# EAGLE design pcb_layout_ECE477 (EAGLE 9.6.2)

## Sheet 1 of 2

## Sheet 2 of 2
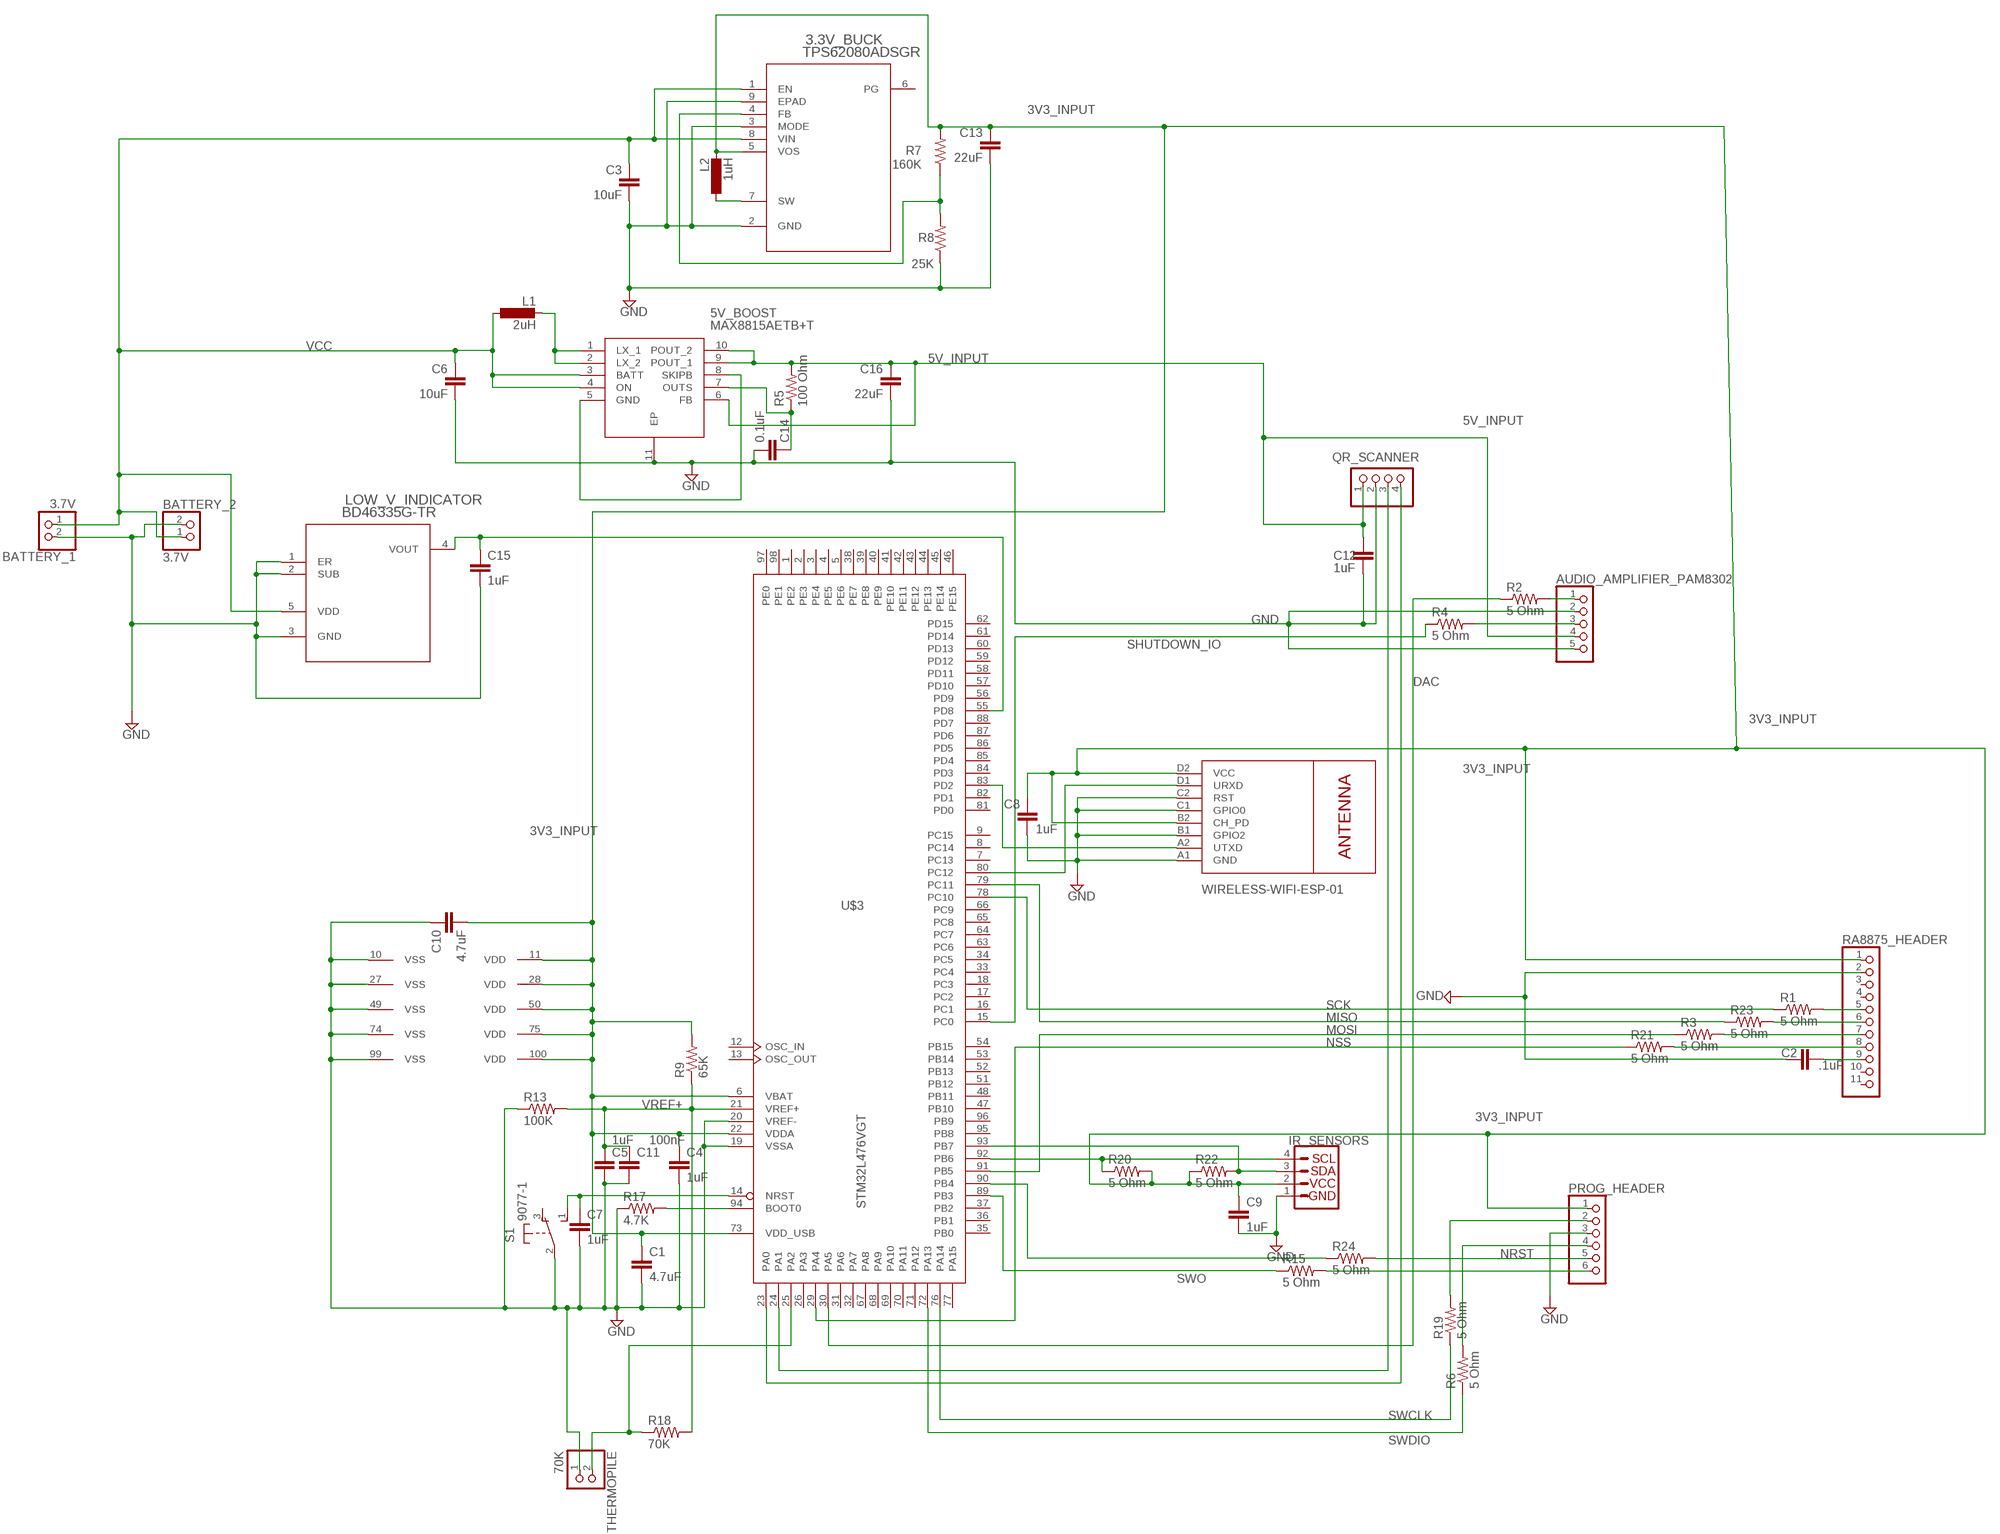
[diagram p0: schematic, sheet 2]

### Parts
3.3V_BUCK  TPS62080ADSGR  [DSG8_1P6X0P9_TEX]
5V_BOOST  MAX8815AETB+T  [SON50P300X300X80-11N]
AUDIO_AMPLIFIER_PAM8302  PINHD-1X5  [1X05]
BATTERY_1  3.7V  JST_2PIN-SMT  [JST-PH-2-SMT]
BATTERY_2  3.7V  JST_2PIN-SMT  [JST-PH-2-SMT]
C1  4.7uF  C2.5/2  [C2.5-2]
C2  .1uF  C2.5/2  [C2.5-2]
C3  10uF  C2.5/2  [C2.5-2]
C4  1uF  C2.5/2  [C2.5-2]
C5  1uF  C2.5/2  [C2.5-2]
C6  10uF  C2.5/2  [C2.5-2]
C7  1uF  C2.5/2  [C2.5-2]
C8  1uF  C2.5/2  [C2.5-2]
C9  1uF  C2.5/2  [C2.5-2]
C10  4.7uF  C2.5/2  [C2.5-2]
C11  100nF  C2.5/2  [C2.5-2]
C12  1uF  C2.5/2  [C2.5-2]
C13  22uF  C2.5/2  [C2.5-2]
C14  0.1uF  C2.5/2  [C2.5-2]
C15  1uF  C2.5/2  [C2.5-2]
C16  22uF  C2.5/2  [C2.5-2]
IR_SENSORS  QWIIC_CONNECTORJS-1MM  [1X04_1MM_RA]
L1  2uH  L-EUIR-4  [IR-4]
L2  1uH  L-EUIR-4  [IR-4]
LOW_V_INDICATOR  BD46335G-TR  [SSOP5_ROM]
PROG_HEADER  PINHD-1X6  [1X06]
QR_SCANNER  PINHD-1X4  [1X04]
R1  5 Ohm  R-US_0309/12  [0309/12]
R2  5 Ohm  R-US_0309/12  [0309/12]
R3  5 Ohm  R-US_0309/12  [0309/12]
R4  5 Ohm  R-US_0309/12  [0309/12]
R5  100 Ohm  R-US_0309/12  [0309/12]
R6  5 Ohm  R-US_0309/12  [0309/12]
R7  160K  R-US_0309/12  [0309/12]
R8  25K  R-US_0309/12  [0309/12]
R9  65K  R-US_0309/12  [0309/12]
R13  100K  R-US_0309/12  [0309/12]
R15  5 Ohm  R-US_0309/12  [0309/12]
R17  4.7K  R-US_0309/12  [0309/12]
R18  70K  R-US_0309/12  [0309/12]
R19  5 Ohm  R-US_0309/12  [0309/12]
R20  5 Ohm  R-US_0309/12  [0309/12]
R21  5 Ohm  R-US_0309/12  [0309/12]
R22  5 Ohm  R-US_0309/12  [0309/12]
R23  5 Ohm  R-US_0309/12  [0309/12]
R24  5 Ohm  R-US_0309/12  [0309/12]
RA8875_HEADER  PINHD-1X11  [1X11]
S1  9077-1  [9077-1]
THERMOPILE  70K  JST_2PIN-SMT  [JST-PH-2-SMT]
U$3  STM32L476VGT  [LQFP100]
U$4  WIRELESS-WIFI-ESP-01  [WIRELESS-WIFI-ESP-01]

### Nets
3V3_INPUT: 3.3V_BUCK.5(VOS) C1.1 C4.1 C8.1 C9.1 C10.2 C13.1 IR_SENSORS.2(VCC) L2.2 PROG_HEADER.1 R7.2 R9.2 R20.2 R22.1 RA8875_HEADER.1 U$3.6(VBAT) U$3.11(VDD) U$3.22(VDDA) U$3.28(VDD) U$3.50(VDD) U$3.73(VDD_USB) U$3.75(VDD) U$3.100(VDD) U$4.B2(CH_PD) U$4.D2(VCC)
5V_INPUT: 5V_BOOST.6(FB) 5V_BOOST.9(POUT_1) 5V_BOOST.10(POUT_2) AUDIO_AMPLIFIER_PAM8302.4 C12.2 C16.1 QR_SCANNER.1 R5.2
DAC: R2.1 U$3.30(PA5)
GND: 3.3V_BUCK.2(GND) 3.3V_BUCK.3(MODE) 3.3V_BUCK.9(EPAD) 5V_BOOST.11(EP) AUDIO_AMPLIFIER_PAM8302.2 AUDIO_AMPLIFIER_PAM8302.5 BATTERY_1.2 BATTERY_2.2 C1.2 C2.1 C3.2 C4.2 C5.2 C6.2 C7.2 C8.2 C9.2 C10.1 C11.2 C12.1 C13.2 C14.2 C15.2 C16.2 IR_SENSORS.1(GND) LOW_V_INDICATOR.1(ER) LOW_V_INDICATOR.2(SUB) LOW_V_INDICATOR.3(GND) PROG_HEADER.3 QR_SCANNER.2 R8.1 R13.1 R17.1 RA8875_HEADER.2 S1.2(P) THERMOPILE.1 U$3.10(VSS) U$3.19(VSSA) U$3.20(VREF-) U$3.27(VSS) U$3.49(VSS) U$3.74(VSS) U$3.99(VSS) U$4.A1(GND) U$4.B1(GPIO2) U$4.C1(GPIO0) U$4.C2(RST)
MISO: R23.1 U$3.79(PC11)
MOSI: R3.1 U$3.91(PB5)
N$1: R17.2 U$3.94(BOOT0)
N$2: C7.1 S1.1(S) U$3.14(NRST)
N$3: PROG_HEADER.4 R6.2
N$4: R18.1 THERMOPILE.2 U$3.25(PA2)
N$5: 3.3V_BUCK.4(FB) R7.1 R8.2
N$6: AUDIO_AMPLIFIER_PAM8302.1 R2.2
N$7: U$3.83(PD2) U$4.A2(UTXD)
N$8: PROG_HEADER.2 R19.2
N$9: 5V_BOOST.1(LX_1) 5V_BOOST.2(LX_2) L1.2
N$10: R24.1 U$3.90(PB4)
N$11: AUDIO_AMPLIFIER_PAM8302.3 R4.2
N$12: R21.2 RA8875_HEADER.8
N$13: C2.2 RA8875_HEADER.9
N$14: PROG_HEADER.6 R15.2
N$15: R3.2 RA8875_HEADER.7
N$16: U$3.80(PC12) U$4.D1(URXD)
N$17: R23.2 RA8875_HEADER.6
N$18: R1.2 RA8875_HEADER.5
N$19: 5V_BOOST.5(GND) 5V_BOOST.8(SKIPB)
N$20: 5V_BOOST.7(OUTS) C14.1 R5.1
N$21: IR_SENSORS.4(SCL) R20.1 U$3.92(PB6)
N$22: IR_SENSORS.3(SDA) R22.2 U$3.93(PB7)
N$23: 3.3V_BUCK.7(SW) L2.1
N$25: C15.1 LOW_V_INDICATOR.4(VOUT) U$3.55(PD8)
N$33: QR_SCANNER.3 U$3.24(PA1)
N$35: QR_SCANNER.4 U$3.23(PA0)
NRST: PROG_HEADER.5 R24.2
NSS: R21.1 U$3.29(PA4)
SCK: R1.1 U$3.78(PC10)
SHUTDOWN_IO: R4.1 U$3.15(PC0)
SWCLK: R19.1 U$3.76(PA14)
SWDIO: R6.1 U$3.72(PA13)
SWO: R15.1 U$3.89(PB3)
VCC: 3.3V_BUCK.1(EN) 3.3V_BUCK.8(VIN) 5V_BOOST.3(BATT) 5V_BOOST.4(ON) BATTERY_1.1 BATTERY_2.1 C3.1 C6.1 L1.1 LOW_V_INDICATOR.5(VDD)
VREF+: C5.1 C11.1 R9.1 R13.2 R18.2 U$3.21(VREF+)
Unconnected: 3.3V_BUCK.6(PG) RA8875_HEADER.3 RA8875_HEADER.4 RA8875_HEADER.10 RA8875_HEADER.11 S1.3(O) U$3.1(PE2) U$3.2(PE3) U$3.3(PE4) U$3.4(PE5) U$3.5(PE6) U$3.7(PC13) U$3.8(PC14) U$3.9(PC15) U$3.12(OSC_IN) U$3.13(OSC_OUT) U$3.16(PC1) U$3.17(PC2) U$3.18(PC3) U$3.26(PA3) U$3.31(PA6) U$3.32(PA7) U$3.33(PC4) U$3.34(PC5) U$3.35(PB0) U$3.36(PB1) U$3.37(PB2) U$3.38(PE7) U$3.39(PE8) U$3.40(PE9) U$3.41(PE10) U$3.42(PE11) U$3.43(PE12) U$3.44(PE13) U$3.45(PE14) U$3.46(PE15) U$3.47(PB10) U$3.48(PB11) U$3.51(PB12) U$3.52(PB13) U$3.53(PB14) U$3.54(PB15) U$3.56(PD9) U$3.57(PD10) U$3.58(PD11) U$3.59(PD12) U$3.60(PD13) U$3.61(PD14) U$3.62(PD15) U$3.63(PC6) U$3.64(PC7) U$3.65(PC8) U$3.66(PC9) U$3.67(PA8) U$3.68(PA9) U$3.69(PA10) U$3.70(PA11) U$3.71(PA12) U$3.77(PA15) U$3.81(PD0) U$3.82(PD1) U$3.84(PD3) U$3.85(PD4) U$3.86(PD5) U$3.87(PD6) U$3.88(PD7) U$3.95(PB8) U$3.96(PB9) U$3.97(PE0) U$3.98(PE1)

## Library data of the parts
3.3V_BUCK = buck_converter:TPS62080ADSGR; BUILT_BY: EMA_UL_Team; MANUFACTURER: Texas Instruments; MANUFACTURER_PART_NUMBER: TPS62080ADSGR; SOURCELIBRARY: TI_2016-07-22; VENDOR: Texas Instruments
5V_BOOST = SamacSys_Parts:MAX8815AETB+T: Boost Switching Regulator IC Positive Adjustable (Fixed) 3.3V (5V) 1 Output 2.75A (Switch) 10-WFDFN Exposed Pad Source: Datasheet; DESCRIPTION: Boost Switching Regulator IC Positive Adjustable (Fixed) 3.3V (5V) 1 Output 2.75A (Switch) 10-WFDFN Exposed Pad; HEIGHT: 0.8mm; MANUFACTURER_NAME: Maxim Integrated; MANUFACTURER_PART_NUMBER: MAX8815AETB+T; MOUSER_PART_NUMBER: 700-MAX8815AETBT; MOUSER_PRICE-STOCK: https://www.mouser.com/Search/Refine.aspx?Keyword=700-MAX8815AETBT
AUDIO_AMPLIFIER_PAM8302 = pinhead:PINHD-1X5: PIN HEADER
BATTERY_1 BATTERY_2 THERMOPILE = adafruit:JST_2PIN: JST 2-Pin Connectors of various flavors
C1-C16 = capacitor-wima:C: CAPACITOR
IR_SENSORS = SparkFun-Connectors:QWIIC_CONNECTOR: SparkFun I2C Standard Qwiic Connector An SMD 1mm pitch JST connector makes it easy and quick (get it? Qwiic?) to connect I2C devices to each other. The Qwiic system enables fast and solderless connection between popular platforms and various sensors and actuators. We carry 200mm, 100mm, 50mm, and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
L1 L2 = rcl:L-EU: INDUCTOR, European symbol; SPICEPREFIX: L
LOW_V_INDICATOR = low_V_IC:BD46335G-TR; BUILT_BY: EMA_Molly; COPYRIGHT: Copyright (C) 2018 Accelerated Designs. All rights reserved; MANUFACTURER_PART_NUMBER: BD46335G-TR; SOURCELIBRARY: ROHM_2019-10-21; VENDOR: ROHM Semiconductor
PROG_HEADER = pinhead:PINHD-1X6: PIN HEADER
QR_SCANNER = pinhead:PINHD-1X4: PIN HEADER
R1-R9 R13 R15 R17-R24 = adafruit:R-US_: RESISTOR, American symbol
RA8875_HEADER = pinhead:PINHD-1X11: PIN HEADER
S1 = switch-misc:9077-1: MARQUARDT SWITCH 9077.0100 Distributor: Buerklin
U$3 = micro-stm_v3:STM32L476V*T: ARM 32-bit Cortex™-M4 CPU 80 MHz maximum frequency 256..1024 Kbytes of Flash memory 128 kbytes of SRAM 82 GPIOs 1.71 to 3.6 V application supply
U$4 = diy-modules:WIRELESS-WIFI-ESP-01: Wireless Wi-Fi ESP-01 Module based on ESP8266 chip Click here to find device on ebay.com

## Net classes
0 test: width 0.305 mm, drill 0.508 mm, clearance 0.127 mm

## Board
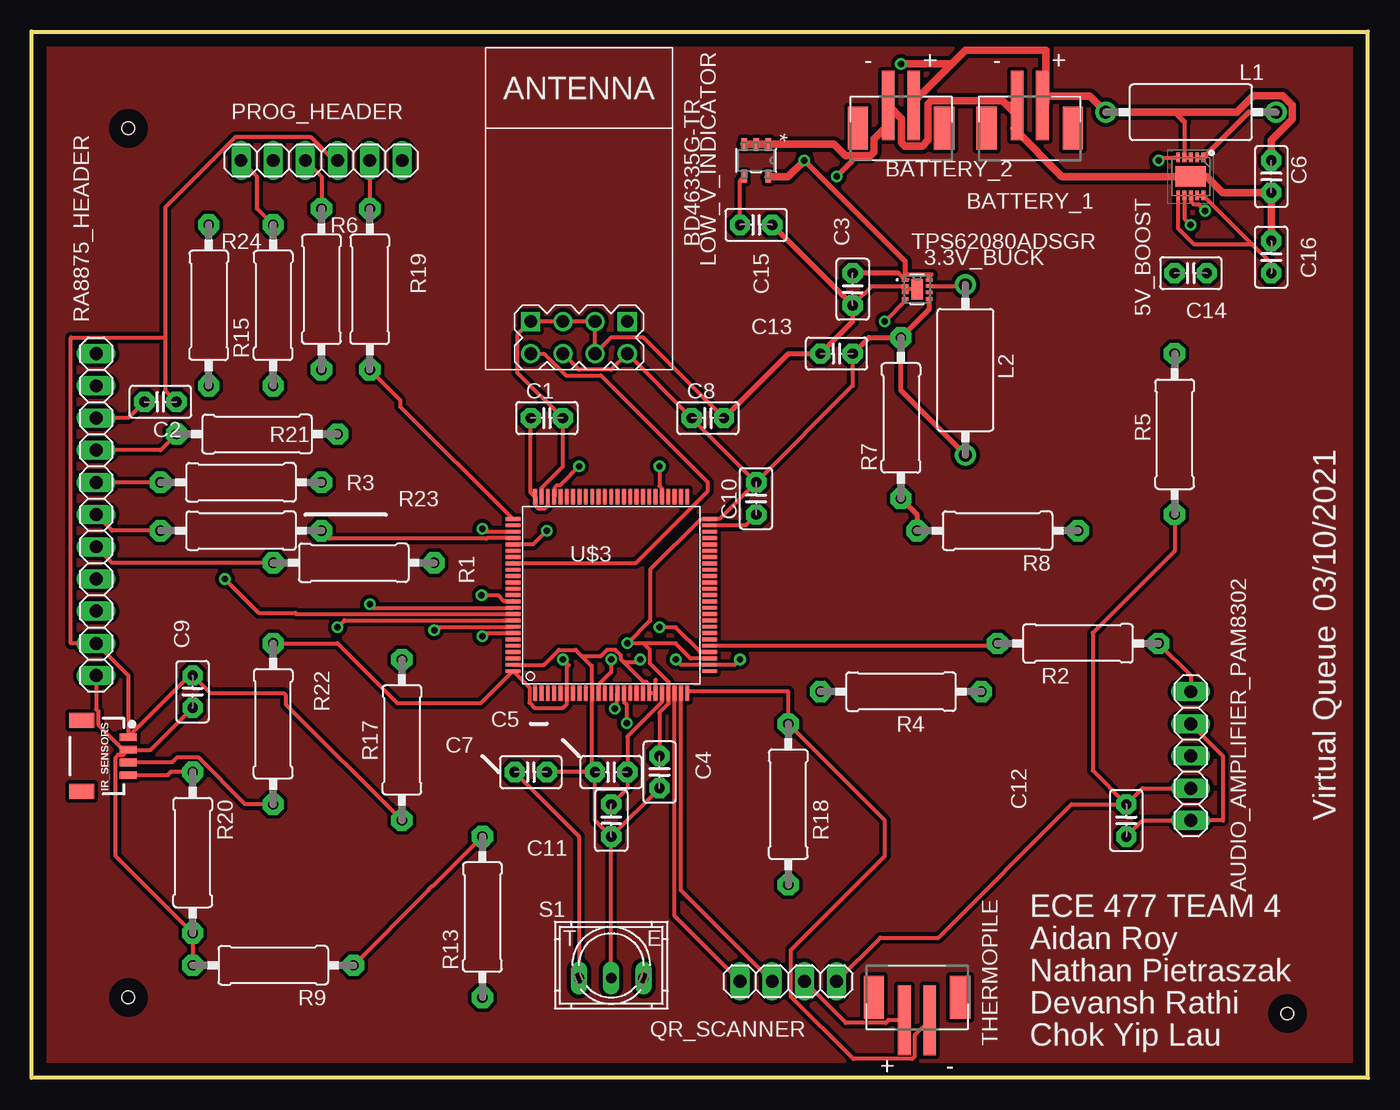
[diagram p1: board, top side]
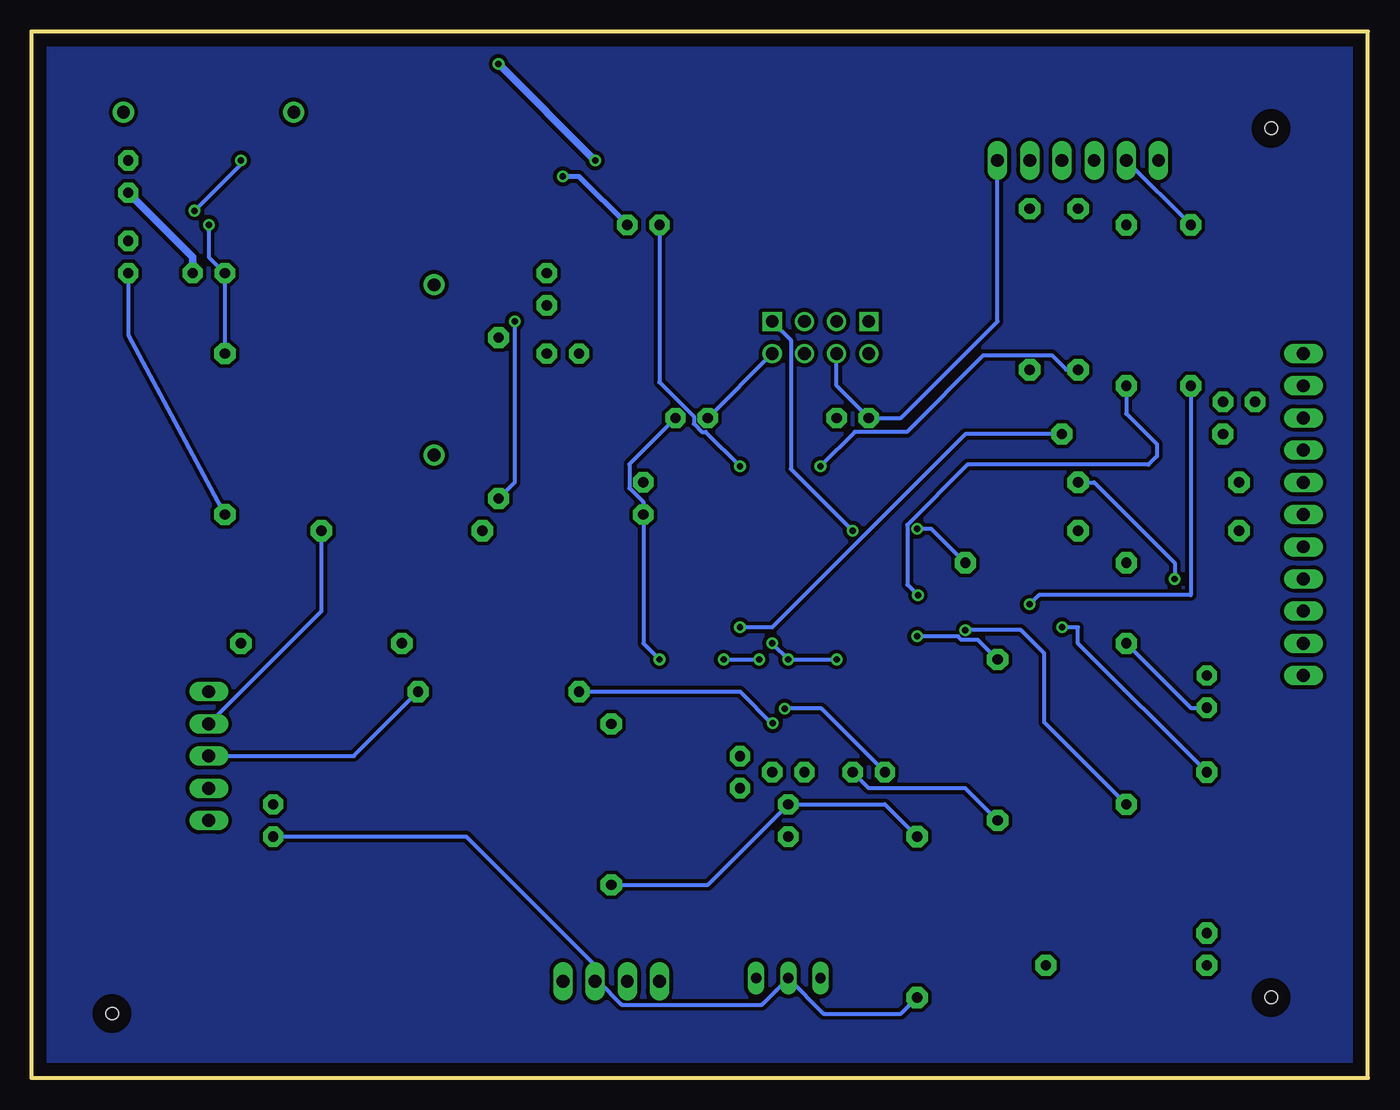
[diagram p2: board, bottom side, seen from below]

Size 105.41 x 82.55 mm. Coordinates in mm from the lower left corner, seen from the top.
Outline: 0,0 0,82.55 105.41,82.55 105.41,0 0,0
Copper layers (1*16): Top 0.035mm / dielectric 1.5mm / Bottom 0.035mm
Design rules "default": minimum track width 6mil, minimum drill 0.35mm, track to track 6mil, track to pad 6mil, pad to pad 6mil, via to via 6mil, smd to smd 6mil, copper to edge 40mil, drill to drill 6mil, minimum pad ring 10mil, minimum via ring 8mil, stop-mask expansion 4mil, vias tented up to drill 0mil, thermal gap 10mil
Holes 1 mm at 7.62,6.35 99.06,5.08 7.62,74.93

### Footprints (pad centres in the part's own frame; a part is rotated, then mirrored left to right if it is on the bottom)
DSG8_1P6X0P9_TEX = smd 0.5 x 0.28: 1 -0.95,0.75; 2 -0.95,0.25; 3 -0.95,-0.25; 4 -0.95,-0.75; 5 0.95,-0.75; 6 0.95,-0.25; 7 0.95,0.25; 8 0.95,0.75 | smd 0.9 x 1.6: 9 0,0
SON50P300X300X80-11N = smd 0.75 x 0.3: 1 -1.5,1; 2 -1.5,0.5; 3 -1.5,0; 4 -1.5,-0.5; 5 -1.5,-1; 6 1.5,-1; 7 1.5,-0.5; 8 1.5,0; 9 1.5,0.5; 10 1.5,1 | smd 1.6 x 2.4: 11 0,0
1X05 = drill 1.016 long: 1 -5.08,0; 2 -2.54,0; 3 0,0; 4 2.54,0; 5 5.08,0
JST-PH-2-SMT = smd 1 x 5.5: 1 -1,-1.8; 2 1,-1.8 | smd 1.6 x 3.4: NC1 -3.4,0; NC2 3.4,0
C2.5-2 = drill 0.813 pad 1.6 octagon: 1 -1.27,0; 2 1.27,0
1X04_1MM_RA = smd 0.6 x 1.35: 1 -1.5,0; 2 -0.5,0; 3 0.5,0; 4 1.5,0 | smd 1.2 x 2: NC1 2.8,-3.675; NC2 -2.8,-3.675
IR-4 = drill 1 pad 1.676: 1 -6.705,0; 2 6.73,0
SSOP5_ROM = smd 0.914 x 0.432: 1 -1.295,0.94; 2 -1.295,0; 3 -1.295,-0.94; 4 1.295,-0.953; 5 1.295,0.953
1X06 = drill 1.016 long: 1 -6.35,0; 2 -3.81,0; 3 -1.27,0; 4 1.27,0; 5 3.81,0; 6 6.35,0
1X04 = drill 1.016 long: 1 -3.81,0; 2 -1.27,0; 3 1.27,0; 4 3.81,0
0309/12 = drill 0.813 pad 1.676 octagon: 1 -6.35,0; 2 6.35,0
1X11 = drill 1.016 long: 1 -12.7,0; 2 -10.16,0; 3 -7.62,0; 4 -5.08,0; 5 -2.54,0; 6 0,0; 7 2.54,0; 8 5.08,0; 9 7.62,0; 10 10.16,0; 11 12.7,0
9077-1 = drill 0.813 long: 1 -2.54,-1.016; 2 0,-1.016; 3 2.54,-1.016
LQFP100 = smd 0.3 x 1.2: 1 -6,-7.75; 2 -5.5,-7.75; 3 -5,-7.75; 4 -4.5,-7.75; 5 -4,-7.75; 6 -3.5,-7.75; 7 -3,-7.75; 8 -2.5,-7.75; 9 -2,-7.75; 10 -1.5,-7.75; 11 -1,-7.75; 12 -0.5,-7.75; 13 0,-7.75; 14 0.5,-7.75; 15 1,-7.75; 16 1.5,-7.75; 17 2,-7.75; 18 2.5,-7.75; 19 3,-7.75; 20 3.5,-7.75; 21 4,-7.75; 22 4.5,-7.75; 23 5,-7.75; 24 5.5,-7.75; 25 6,-7.75; 51 6,7.75; 52 5.5,7.75; 53 5,7.75; 54 4.5,7.75; 55 4,7.75; 56 3.5,7.75; 57 3,7.75; 58 2.5,7.75; 59 2,7.75; 60 1.5,7.75; 61 1,7.75; 62 0.5,7.75; 63 0,7.75; 64 -0.5,7.75; 65 -1,7.75; 66 -1.5,7.75; 67 -2,7.75; 68 -2.5,7.75; 69 -3,7.75; 70 -3.5,7.75; 71 -4,7.75; 72 -4.5,7.75; 73 -5,7.75; 74 -5.5,7.75; 75 -6,7.75 | smd 1.2 x 0.3: 26 7.75,-6; 27 7.75,-5.5; 28 7.75,-5; 29 7.75,-4.5; 30 7.75,-4; 31 7.75,-3.5; 32 7.75,-3; 33 7.75,-2.5; 34 7.75,-2; 35 7.75,-1.5; 36 7.75,-1; 37 7.75,-0.5; 38 7.75,0; 39 7.75,0.5; 40 7.75,1; 41 7.75,1.5; 42 7.75,2; 43 7.75,2.5; 44 7.75,3; 45 7.75,3.5; 46 7.75,4; 47 7.75,4.5; 48 7.75,5; 49 7.75,5.5; 50 7.75,6; 76 -7.75,6; 77 -7.75,5.5; 78 -7.75,5; 79 -7.75,4.5; 80 -7.75,4; 81 -7.75,3.5; 82 -7.75,3; 83 -7.75,2.5; 84 -7.75,2; 85 -7.75,1.5; 86 -7.75,1; 87 -7.75,0.5; 88 -7.75,0; 89 -7.75,-0.5; 90 -7.75,-1; 91 -7.75,-1.5; 92 -7.75,-2; 93 -7.75,-2.5; 94 -7.75,-3; 95 -7.75,-3.5; 96 -7.75,-4; 97 -7.75,-4.5; 98 -7.75,-5; 99 -7.75,-5.5; 100 -7.75,-6
WIRELESS-WIFI-ESP-01 = drill 1 square: A1 -8.89,3.81; D1 -8.89,-3.81 | drill 1: A2 -11.43,3.81; B1 -8.89,1.27; B2 -11.43,1.27; C1 -8.89,-1.27; C2 -11.43,-1.27; D2 -11.43,-3.81

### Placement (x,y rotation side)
3.3V_BUCK  69.85,62.23 0 top
5V_BOOST  91.44,71.12 270 top
AUDIO_AMPLIFIER_PAM8302  91.44,25.4 270 top
BATTERY_1  78.74,74.93 180 top
BATTERY_2  68.58,74.93 180 top
C1  40.64,52.07 0 top
C2  10.16,53.34 180 top
C3  64.77,62.23 270 top
C4  49.53,24.13 270 top
C5  45.72,24.13 180 top
C6  97.79,71.12 270 top
C7  39.37,24.13 0 top
C8  53.34,52.07 0 top
C9  12.7,30.48 90 top
C10  57.15,45.72 90 top
C11  45.72,20.32 270 top
C12  86.36,20.32 90 top
C13  63.5,57.15 180 top
C14  91.44,63.5 0 top
C15  57.15,67.31 0 top
C16  97.79,64.77 90 top
IR_SENSORS  7.62,25.4 270 top
L1  91.44,76.2 0 top
L2  73.66,55.88 270 top
LOW_V_INDICATOR  57.15,72.39 270 top
PROG_HEADER  22.86,72.39 180 top
QR_SCANNER  59.69,7.62 180 top
R1  25.4,40.64 180 top
R2  82.55,34.29 0 top
R3  16.51,46.99 180 top
R4  68.58,30.48 0 top
R5  90.17,50.8 270 top
R6  22.86,62.23 90 top
R7  68.58,52.07 90 top
R8  76.2,43.18 180 top
R9  19.05,8.89 180 top
R13  35.56,12.7 90 top
R15  19.05,60.96 90 top
R17  29.21,26.67 90 top
R18  59.69,21.59 270 top
R19  26.67,62.23 90 top
R20  12.7,17.78 270 top
R21  17.78,50.8 180 top
R22  19.05,27.94 270 top
R23  16.51,43.18 180 top
R24  13.97,60.96 90 top
RA8875_HEADER  5.08,44.45 90 top
S1  45.72,8.89 0 top
THERMOPILE  69.85,6.35 0 top
U$3  45.72,38.1 0 top
U$4  43.18,68.58 90 top

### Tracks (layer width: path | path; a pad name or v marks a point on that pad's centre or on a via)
3V3_INPUT  (via drill 0.51)
  Top 0.305: C4.1 49.53,28.83 50.22,29.52 | C1.1 39.37,46.2 U$3.75 39.76,45.81 39.76,45.13 39.94,44.95 40.5,44.95 40.72,45.17 U$3.73 | C10.2 54.26,44.1 U$3.50 53.43,44.06 52.75,44.06 48.79,40.11 48.79,36.09 v46.99,34.29 48.26,34.29 | U$4.B2 43.18,55.88 45.72,55.88 U$4.D2 C8.1 C10.2 | RA8875_HEADER.1 5.08,29.1 5.25,28.93 5.25,27.86 7.21,25.9 IR_SENSORS.2 | IR_SENSORS.2 9.39,25.9 C9.1 | IR_SENSORS.2 7.22,25.5 6.82,25.5 6.64,25.33 6.64,17.49 R20.2 R9.2 | U$3.11 44.72,30.88 44.77,30.93 44.77,31.08 45.72,32.03 v45.72,33.02 | U$3.22 50.22,29.52 | 50.22,29.52 50.26,29.56 50.26,31.21 48.77,32.7 48.77,33.78 48.26,34.29 | U$3.28 51.99,33.1 50.8,34.29 48.26,34.29 | v41.91,33.02 42.35,32.58 42.22,32.44 U$3.6 42.22,29.52 41.91,29.21 39.68,29.21 39.27,29.62 39.27,30.8 U$3.100 35.43,29.56 28.86,29.56 24.13,34.29 R22.1 | C13.1 64.77,54.61 C10.2
  Top 0.406: 3.3V_BUCK.5 70.8,60.64 R7.2 | C13.1 66.04,58.42 R7.2 | L2.2 68.58,54.23 R7.2
  Bottom 0.305: C8.1 U$4.D2 | U$4.B2 41.91,54.61 C1.1 36.83,52.07 29.21,59.69 PROG_HEADER.1 | v41.91,33.02 v45.72,33.02 v46.99,34.29 | R22.1 13.97,29.21 C9.1
5V_INPUT
  Top 0.305: QR_SCANNER.1 66.95,11.07 71.52,11.07 82.03,21.59 C12.2 | C12.2 87.63,22.86 AUDIO_AMPLIFIER_PAM8302.4 | C12.2 83.7,24.25 83.7,35.12 90.17,41.59 R5.2 | 5V_BOOST.9 5V_BOOST.10 96.27,65.79 | C16.1 97.79,64.27 96.27,65.79 | 5V_BOOST.6 90.44,67.04 91.69,65.79 96.27,65.79
  Bottom 0.305: C16.1 97.79,58.6 R5.2
COPPER_POURS_1
  pour Top (isolate 0.305): 0,82.55 0,0 105.41,0 105.41,82.55
COPPER_POURS_16
  pour Bottom (isolate 0.305): 0,82.55 0,0 105.41,0 105.41,82.55
DAC
  Top 0.305: U$3.30 73.66,34.1 73.85,34.1 76.01,34.1 R2.1
GND  (via drill 0.51)
  Top 0.305: C4.2 C11.2 | C11.2 44.45,20.32 C5.2 | S1.2 C11.2 | C10.1 56.3,43.6 U$3.49 | C8.2 48.26,58.42 45.72,58.42 U$4.C2 U$4.C1 U$4.B1 U$4.A1 38.31,58.63 38.31,55.67 C1.2 41.91,48.22 40.22,46.53 U$3.74 | PROG_HEADER.3 23.86,72.39 22.03,74.22 16.07,74.22 10.54,68.7 10.54,58.42 | 10.54,58.42 10.54,54.23 C2.1 | 10.54,58.42 3.1,58.42 3.1,34.29 RA8875_HEADER.2 7.62,31.75 IR_SENSORS.1 12.47,31.75 C9.2 14.09,30.36 19.88,30.36 20.05,30.18 20.05,29.47 R17.1 | 44.17,31.08 44.17,30.39 U$3.10 44.22,24.36 C5.2 | 44.17,31.08 44.27,31.08 | C5.2 C7.2 | 44.17,31.08 44.17,32.52 43.43,33.27 | v55.88,33.02 55.46,32.6 U$3.27 51.22,32.6 v50.8,33.02 | U$3.20 U$3.19 | U$3.19 48.72,31.03 48.5,31.25 48.26,31.25 46.74,32.77 | U$3.19 U$3.20 49.22,31.44 | U$3.99 40.41,32.6 41.59,33.78 42.92,33.78 43.43,33.27 | 46.74,32.77 46.48,33.03 46.48,33.34 46.04,33.78 45.4,33.78 44.89,33.27 43.43,33.27 | v48.01,33.02 47.76,32.77 46.74,32.77 | C12.1 87.63,20.32 AUDIO_AMPLIFIER_PAM8302.5 93.98,20.32 93.98,25.4 AUDIO_AMPLIFIER_PAM8302.2 | 5V_BOOST.11 92.71,71.12 | C3.2 66.28,62.47 68.58,62.47 68.9,62.15 3.3V_BUCK.3 | 3.3V_BUCK.9 69.15,62.23 3.3V_BUCK.2 3.3V_BUCK.3 | 3.3V_BUCK.2 3.3V_BUCK.3 | THERMOPILE.1 67.58,4.55 67.38,4.34 64.23,4.34 QR_SCANNER.2
  Top 0.406: v63.5,71.12 64.77,72.39 64.77,72.77 | C15.2 C3.2 64.77,59.69 C13.2 59.69,57.15 C8.2
  Top 0.61: 76.94,76.73 76.58,77.09 70.99,77.09 70.72,76.82 70.72,73.98 70.27,73.52 68.89,73.52 68.62,73.79 68.62,75.69 BATTERY_2.2 67.58,75.2 66.44,74.06 66.44,73.04 66.17,72.77 64.77,72.77 64.19,72.77 63.28,73.69 LOW_V_INDICATOR.1 LOW_V_INDICATOR.2 LOW_V_INDICATOR.3 | 76.94,76.73 77.47,76.2 | 92.71,71.12 93.98,69.85 C6.2 C16.2 | 5V_BOOST.11 81.28,71.12 77.47,74.93 77.74,75.2 BATTERY_1.2 76.94,76.73
  Bottom 0.305: C7.2 39.37,22.86 31.75,22.86 R17.1 | v55.88,33.02 57.15,34.29 C10.1 57.15,45.43 58.26,46.53 58.26,48.42 C8.2 | v50.8,33.02 v48.01,33.02 | C12.1 71.12,19.05 60.96,8.89 QR_SCANNER.2 60.69,7.62 58.86,5.79 47.8,5.79 S1.2 42.93,5.08 36.83,5.08 R13.1 | AUDIO_AMPLIFIER_PAM8302.2 82.55,36.83 R8.1
  Bottom 0.406: C15.2 62.23,71.12 v63.5,71.12
  Bottom 0.61: C6.2 92.71,64.77 C14.2
MISO
  Top 0.305: U$3.79 35.92,42.6 35.88,42.56 23.48,42.56 R23.1
MOSI  (via drill 0.51)
  Top 0.305: U$3.91 20.9,36.6 20.79,36.7 17.91,36.7 v15.24,39.37
  Bottom 0.305: v15.24,39.37 15.24,40.64 21.59,46.99 R3.1
N$1  (via drill 0.51)
  Top 0.305: v35.56,34.84 35.82,35.1 U$3.94
  Bottom 0.305: v35.56,34.84 32.33,34.84 32.07,34.58 30.77,34.58 R17.2
N$2  (via drill 0.51)
  Top 0.305: U$3.14 46.17,30.3 46.17,29.62 46,29.45 v46,29.14 | C7.1 43.18,19.05 S1.1
  Bottom 0.305: C7.1 43.11,29.14 v46,29.14
N$3
  Top 0.305: PROG_HEADER.4 22.86,71.12 R6.2
N$4
  Top 0.305: U$3.25 51.85,30.48 59.69,30.48 R18.1 67.31,20.32 67.31,17.51 59.89,10.09 59.89,6.42 64.81,1.5 69.48,1.5 69.66,1.67 69.66,3.35 THERMOPILE.2
N$5  (via drill 0.51)
  Top 0.305: 3.3V_BUCK.4 68.9,61.28 v67.31,59.69
  Top 0.406: R7.1 69.85,44.45 R8.2
  Bottom 0.305: v67.31,59.69 67.31,46.99 R7.1
N$6
  Top 0.305: R2.2 91.44,31.75 AUDIO_AMPLIFIER_PAM8302.1
N$7
  Top 0.305: U$3.83 38.02,40.64 47.7,40.64 53.34,46.29 53.34,46.99 44.91,55.42 42.14,55.42 40.41,57.15 U$4.A2
N$8
  Top 0.305: PROG_HEADER.2 R19.2
N$9
  Top 0.305: 5V_BOOST.2 5V_BOOST.1 5V_BOOST.2
  Top 0.406: 5V_BOOST.1 96.02,76.2 L1.2
N$10  (via drill 0.51)
  Top 0.305: v26.67,37.36 26.93,37.1 U$3.90
  Bottom 0.305: v26.67,37.36 25.93,38.1 13.97,38.1 R24.1
N$11
  Bottom 0.305: AUDIO_AMPLIFIER_PAM8302.3 80.01,25.4 R4.2
N$12
  Top 0.305: R21.2 10.16,49.53 RA8875_HEADER.8
N$13
  Top 0.305: C2.2 7.62,52.07 RA8875_HEADER.9
N$14
  Top 0.305: PROG_HEADER.6 17.78,71.12 17.78,68.58 R15.2
N$15
  Top 0.305: R3.2 RA8875_HEADER.7
N$16  (via drill 0.51)
  Top 0.305: v40.64,43.18 39.56,42.1 U$3.80
  Bottom 0.305: v40.64,43.18 45.51,48.05 45.51,58.21 U$4.D1
N$17
  Top 0.305: R23.2 6.35,43.18 RA8875_HEADER.6
N$18
  Top 0.305: R1.2 6.35,40.64 RA8875_HEADER.5
N$19  (via drill 0.51)
  Top 0.305: 5V_BOOST.8 91.48,69.58 91.48,69.12 91.66,68.94 92.04,68.94 v92.56,68.43 | v88.9,72.39 89.13,72.62 90.17,72.62 5V_BOOST.5
  Bottom 0.305: v92.56,68.43 88.9,72.08 v88.9,72.39
N$20  (via drill 0.51)
  Top 0.305: 5V_BOOST.7 90.94,67.81 v91.44,67.31
  Bottom 0.305: v91.44,67.31 91.44,64.77 C14.1 R5.1
N$21  (via drill 0.51)
  Top 0.305: IR_SENSORS.4 10.74,23.9 10.97,24.13 R20.1 | v24.13,35.56 24.67,36.1 U$3.92
  Bottom 0.305: v24.13,35.56 22.86,35.56 22.86,34.29 R20.1
N$22  (via drill 0.51)
  Top 0.305: v31.75,35.34 32.01,35.6 U$3.93 | IR_SENSORS.3 11.1,24.9 11.47,25.27 13.17,25.27 16.86,21.59 R22.2
  Bottom 0.305: v31.75,35.34 27.37,35.34 25.53,33.49 25.53,28.07 R22.2
N$23
  Top 0.305: 3.3V_BUCK.7 73.56,62.48 L2.1
N$25  (via drill 0.51)
  Top 0.305: v49.53,48.26 49.53,46.72 49.67,46.58 49.67,45.89 U$3.55 | C15.1 55.88,70.78 LOW_V_INDICATOR.4
  Bottom 0.305: v49.53,48.26 52.23,50.96 52.53,50.96 53.17,51.61 53.17,52.2 55.88,54.9 C15.1
N$33
  Top 0.305: QR_SCANNER.3 51.22,14.82 U$3.24
N$35
  Top 0.305: QR_SCANNER.4 50.72,12.78 U$3.23
NRST
  Bottom 0.305: PROG_HEADER.5 R24.2
NSS  (via drill 0.51)
  Top 0.305: U$3.29 52.76,33.6 50.8,35.56 v49.53,35.56
  Bottom 0.305: v49.53,35.56 46.99,35.56 31.75,50.8 R21.1
SCK  (via drill 0.51)
  Top 0.305: v35.56,43.32 35.78,43.1 U$3.78
  Bottom 0.305: R1.1 34.43,43.32 v35.56,43.32
SHUTDOWN_IO  (via drill 0.51)
  Top 0.305: U$3.15 46.77,30.3 46.77,29.62 46.95,29.44 v46.95,27.98
  Bottom 0.305: v46.95,27.98 46.99,27.94 49.53,30.48 R4.1
SWCLK
  Top 0.305: U$3.76 29.08,52.99 29.08,53.47 R19.1
SWDIO  (via drill 0.51)
  Top 0.305: U$3.72 41.27,45.89 41.27,46.58 41.44,46.76 41.67,46.76 v43.18,48.26
  Bottom 0.305: v43.18,48.26 40.48,50.96 36.37,50.96 30.31,57.02 24.93,57.02 23.78,55.88 R6.1
SWO  (via drill 0.51)
  Top 0.305: U$3.89 37.92,37.64 37.24,37.64 36.79,38.1 v35.49,38.1
  Bottom 0.305: v35.49,38.1 36.32,38.93 36.32,43.63 31.57,48.39 17.31,48.39 16.64,49.06 16.64,50 17.61,50.97 17.78,51.15 19.05,52.42 R15.1
VCC  (via drill 0.51)
  Top 0.305: 5V_BOOST.3 5V_BOOST.4 90.94,75.43 | 3.3V_BUCK.8 70.8,63.18 71.01,63.39 69.01,63.39 68.9,63.27 3.3V_BUCK.1 68.38,63.5
  Top 0.406: v60.96,72.39 68.9,64.45 68.9,63.5 69.01,63.39 | 68.38,63.5 C3.1 | 90.17,76.2 90.94,75.43
  Top 0.61: 72.49,79.91 73.66,81.08 80.01,81.08 80.01,77.47 | 72.49,79.91 69.58,77 BATTERY_2.1 | 80.01,77.47 80.01,77 BATTERY_1.1 | 80.01,77.47 83.47,77.47 L1.1 90.17,76.2 95.09,76.2 96.38,77.5 98.71,77.5 99.47,76.74 99.47,75.66 97.79,73.99 C6.1 | LOW_V_INDICATOR.5 59.66,71.1 v60.96,72.39 | v68.58,80.01 72.39,80.01 72.49,79.91
  Bottom 0.61: v60.96,72.39 v68.58,80.01
VREF+
  Top 0.305: C11.1 46.99,22.86 C5.1 46.99,26.94 49.72,29.67 U$3.21 | R9.1 31.29,14.78 31.29,14.85 31.56,15.12 31.63,15.12 R13.2
  Bottom 0.305: R13.2 38.1,21.59 C11.1 52.07,15.24 R18.2

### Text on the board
tPlace: 03/10/2021 | Virtual Queue | ECE 477 TEAM 4 | Aidan Roy | Nathan Pietraszak | Devansh Rathi | Chok Yip Lau

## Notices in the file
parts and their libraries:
SparkFun-Connectors: Licensing: Creative Commons ShareAlike 4.0 International - https://creativecommons.org/licenses/by-sa/4.0
diy-modules: Released under the Creative Commons Attribution 4.0 International License: http://creativecommons.org/licenses/by/4.0
